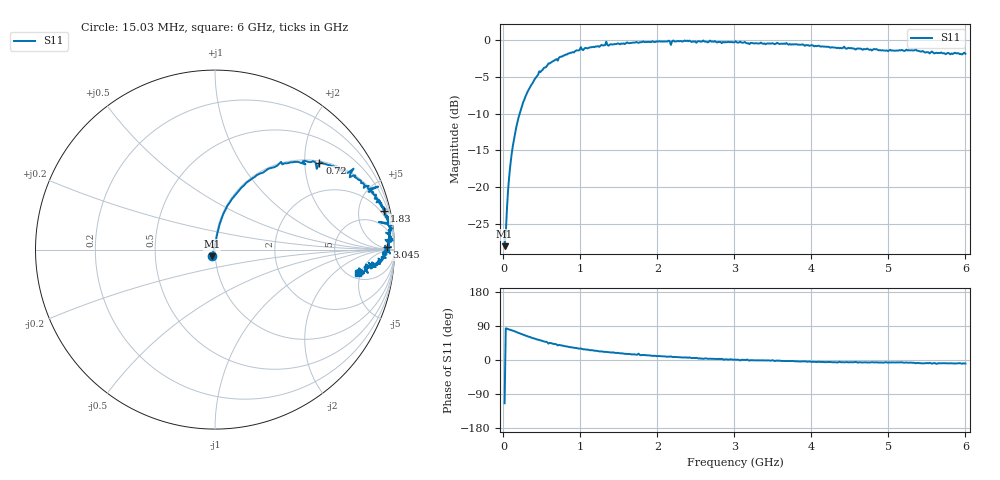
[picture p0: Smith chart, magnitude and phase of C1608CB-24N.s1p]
!	Network	Analyzer	HP8753E.07.74:	Oct	30	2002	Serial	No.	JP38451487
!	Hewlett-Packard
!	28	Aug	2009	16:01:57
!	Frequency	S11
#	HZ	S	RI	R	50
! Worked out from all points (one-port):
!   400 points, 15.03 MHz to 6 GHz, reference 50 ohm
!   lowest |S11| = -28.0 dB at 15.03 MHz (marker M1), VSWR 1.08, Z = 48.3 - j3.51 ohm
!   |S11| at or under -10 dB: start of sweep to 211.6 MHz
!   S11 on the Smith chart (normalised r, x): 15.03 MHz: 0.97, -0.07; 720 MHz: 1.05, +2.37; 1.83 GHz: 1.28, +8.66; 3.045 GHz: 42, +14; 6 GHz: 6.02, -4.38
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1.502992e7  -0.0163 -0.0363
3.002985e7  0.00555 0.048
6.00297e7  0.014 0.0946
9.002955e7  0.0255 0.14
1.95029e8  0.0937 0.281
3.150284e8  0.207 0.396
4.650277e8  0.368 0.489
7.200264e8  0.582 0.483
7.650262e8  0.606 0.479
1.005025e9  0.772 0.451
1.320023e9  0.858 0.338
1.335023e9  0.909 0.351
1.365023e9  0.855 0.322
1.515022e9  0.89 0.284
1.740021e9  0.933 0.235
1.755021e9  0.914 0.276
1.785021e9  0.943 0.209
1.830021e9  0.943 0.216
2.145019e9  0.976 0.152
2.175019e9  0.913 0.154
2.205019e9  0.983 0.134
2.265019e9  0.975 0.13
3.015015e9  0.981 0.014
3.045015e9  0.958 0.0139
3.765011e9  0.929 -0.044
4.515007e9  0.878 -0.0881
5.265004e9  0.846 -0.106
6e9  0.795 -0.128
